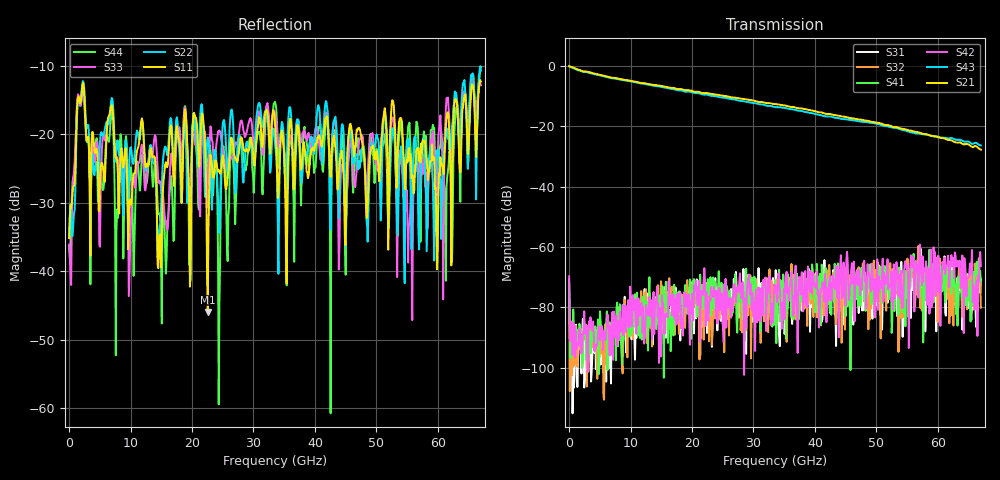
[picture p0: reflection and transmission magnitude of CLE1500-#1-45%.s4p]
!Keysight Technologies,N5247B,US50470101,A.16.20.02
!Date: Thursday, March 13, 2025 10:21:04
!Correction: S11(C  4-Port  )
!S12(C  4-Port  )
!S13(C  4-Port  )
!S14(C  4-Port  )
!S21(C  4-Port  )
!S22(C  4-Port  )
!S23(C  4-Port  )
!S24(C  4-Port  )
!S31(C  4-Port  )
!S32(C  4-Port  )
!S33(C  4-Port  )
!S34(C  4-Port  )
!S41(C  4-Port  )
!S42(C  4-Port  )
!S43(C  4-Port  )
!S44(C  4-Port  )
!S4P File: Measurements: <S11,S12,S13,S14>,
!<S21,S22,S23,S24>,
!<S31,S32,S33,S34>,
!<S41,S42,S43,S44>:
# Hz S  dB  R 50
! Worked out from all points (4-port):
!   601 points, 10 MHz to 67 GHz, reference 50 ohm
!   strongest paths, dB at 10 MHz, 16.76 GHz, 33.51 GHz, 50.25 GHz, 67 GHz:
!     S21: 0.0, -7.2, -12.6, -18.8, -27.7
!     S43: 0.0, -7.5, -13.6, -19.2, -26.3
!     S42: -69.7, -82.7, -75.4, -80.8, -66.3
!     S41: -70.8, -87.6, -71.0, -68.4, -71.4
!     S32: -76.4, -73.1, -73.6, -65.2, -80.1
!     S31: -71.9, -79.4, -81.0, -75.8, -70.6
!   lowest |S11| = -45.9 dB at 22.56 GHz (marker M1), VSWR 1.01, Z = 50.5 + j0.216 ohm
!   |S11| at or under -10 dB: start of sweep to end of sweep
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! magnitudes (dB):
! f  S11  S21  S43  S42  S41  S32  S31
! 10 MHz  -35.1  0.0  0.0  -69.7  -70.8  -76.4  -71.9
! 2.131 GHz  -13.1  -1.6  -1.8  -94.9  -100.0  -90.9  -88.8
! 7.714 GHz  -23.4  -4.0  -4.2  -82.7  -80.4  -90.8  -89.8
! 22.56 GHz  -45.9  -9.0  -9.5  -81.7  -70.6  -75.2  -76.6
! 52.6 GHz  -15.0  -20.0  -20.4  -68.3  -83.6  -67.3  -67.5
! 55.5 GHz  -22.9  -21.4  -21.9  -66.6  -73.7  -70.2  -67.4
! 67 GHz  -12.3  -27.7  -26.3  -66.3  -71.4  -80.1  -70.6
